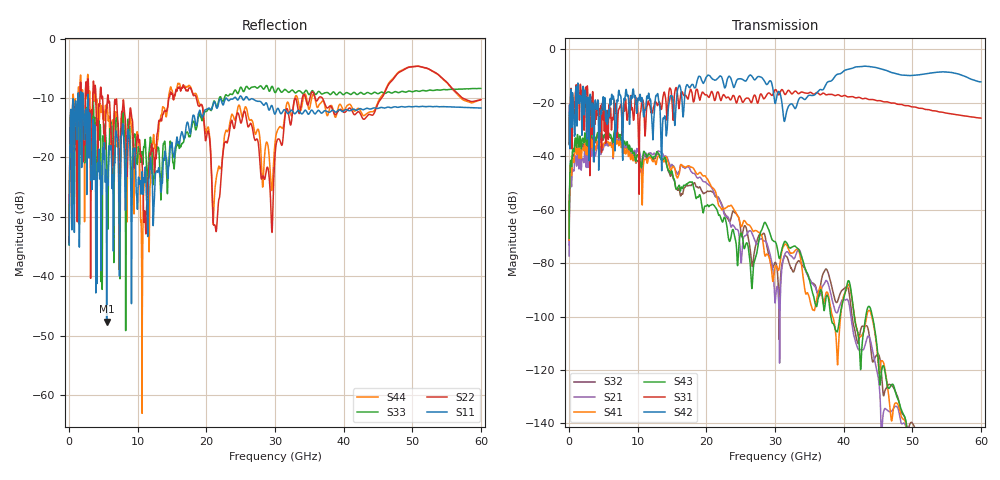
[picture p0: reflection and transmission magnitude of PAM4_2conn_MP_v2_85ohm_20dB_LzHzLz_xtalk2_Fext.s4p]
! Info: Touchstone file created by Circ.  Input file=FAB50GbE_2conn_Midplane_Examax_Topo2_v2_85ohm_20dB_LzHzLz.circ
# Hz S RI R 50
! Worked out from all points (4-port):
!   6000 points, 10 MHz to 60 GHz, reference 50 ohm
!   strongest paths, dB at 10 MHz, 15.01 GHz, 30.01 GHz, 45.01 GHz, 60 GHz:
!     S42: -35.6, -17.4, -20.2, -7.0, -12.1
!     S31: -35.4, -20.1, -15.1, -19.2, -25.7
!     S43: -70.7, -45.8, -71.9, -114.9, -160.9
!     S41: -71.4, -44.2, -81.6, -116.5, -175.6
!     S21: -77.3, -43.1, -95.0, -122.4, -166.8
!     S32: -73.1, -46.4, -79.8, -114.0, -152.9
!   lowest |S11| = -47.7 dB at 5.48 GHz (marker M1), VSWR 1.01, Z = 49.9 - j0.408 ohm
!   |S11| at or under -10 dB: start of sweep to 1.285 GHz; 2.783 GHz to 24.03 GHz (21.24 GHz wide, 158 % of centre); 26 GHz to end of sweep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
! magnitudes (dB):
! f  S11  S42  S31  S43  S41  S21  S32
! 10 MHz  -34.7  -35.6  -35.4  -70.7  -71.4  -77.3  -73.1
! 1.06 GHz  -12.8  -14.0  -13.4  -35.8  -38.5  -42.4  -37.9
! 5.48 GHz  -47.7  -24.5  -29.7  -31.0  -34.1  -34.6  -32.1
! 10.65 GHz  -22.6  -18.2  -18.9  -42.3  -57.7  -46.0  -44.3
! 14.79 GHz  -18.1  -17.4  -14.7  -46.5  -45.5  -44.1  -47.5
! 26.65 GHz  -10.1  -10.0  -19.6  -89.4  -67.3  -68.8  -80.7
! 60 GHz  -11.7  -12.1  -25.7  -160.9  -175.6  -166.8  -152.9
